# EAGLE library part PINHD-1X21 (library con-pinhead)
PIN HEADER
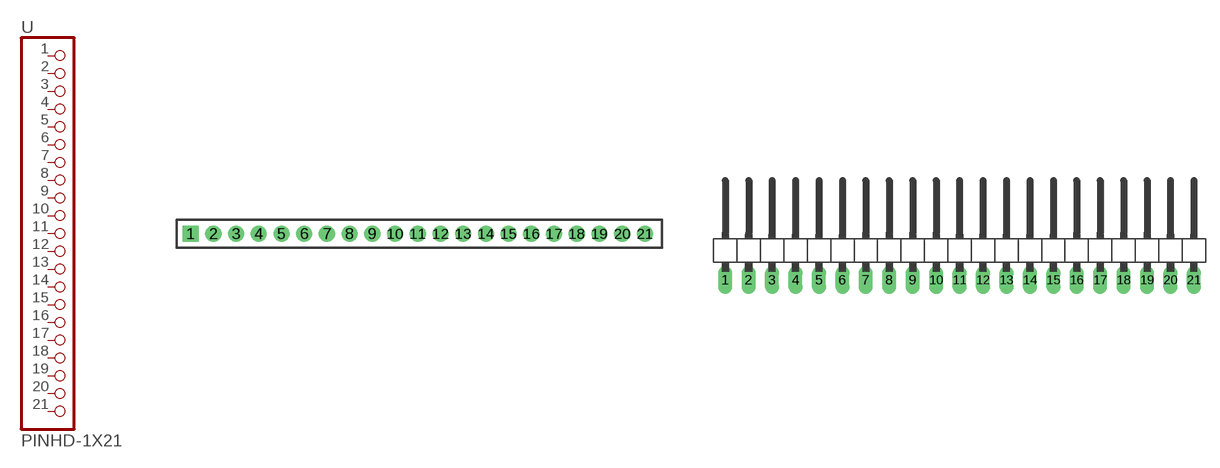
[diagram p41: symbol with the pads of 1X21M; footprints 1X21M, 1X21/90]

Designator prefix -

## PINHD-1X21_2.00  [1X21M]
1  1  pas
2  2  pas
3  3  pas
4  4  pas
5  5  pas
6  6  pas
7  7  pas
8  8  pas
9  9  pas
10  10  pas
11  11  pas
12  12  pas
13  13  pas
14  14  pas
15  15  pas
16  16  pas
17  17  pas
18  18  pas
19  19  pas
20  20  pas
21  21  pas

## PINHD-1X21_2.54-90°  [1X21/90]
Pads as for 1X21M

## PINHD-1X21_2.54  [1X21]
Pads as for 1X21M

## PINHD-1X21_2.54-SMD  [1X21SMD]
Pads as for 1X21M

## PINHD-1X21_2.54-SMD-90°  [1X21SMD/90]
Pads as for 1X21M

## Footprint 1X21M (pad centres in mm)
PIN HEADER - 2
drill 0.914 square: 1 -19,0
drill 0.914: 2 -17,0; 3 -15,0; 4 -13,0; 5 -11,0; 6 -9,0; 7 -7,0; 8 -5,0; 9 -3,0; 10 -1,0; 11 1,0; 12 3,0; 13 5,0; 14 7,0; 15 9,0; 16 11,0; 17 13,0; 18 15,0; 19 17,0; 20 19,0; 21 21,0

## Footprint 1X21/90 (pad centres in mm)
PIN HEADER - 2.54 90°
drill 1.016 long: 1 -24.13,-3.81; 2 -21.59,-3.81; 3 -19.05,-3.81; 4 -16.51,-3.81; 5 -13.97,-3.81; 6 -11.43,-3.81; 7 -8.89,-3.81; 8 -6.35,-3.81; 9 -3.81,-3.81; 10 -1.27,-3.81; 11 1.27,-3.81; 12 3.81,-3.81; 13 6.35,-3.81; 14 8.89,-3.81; 15 11.43,-3.81; 16 13.97,-3.81; 17 16.51,-3.81; 18 19.05,-3.81; 19 21.59,-3.81; 20 24.13,-3.81; 21 26.67,-3.81

## Footprint 1X21 (pad centres in mm)
PIN HEADER - 2.54
drill 1.016 long: 1 -24.13,0; 2 -21.59,0; 3 -19.05,0; 4 -16.51,0; 5 -13.97,0; 6 -11.43,0; 7 -8.89,0; 8 -6.35,0; 9 -3.81,0; 10 -1.27,0; 11 1.27,0; 12 3.81,0; 13 6.35,0; 14 8.89,0; 15 11.43,0; 16 13.97,0; 17 16.51,0; 18 19.05,0; 19 21.59,0; 20 24.13,0; 21 26.67,0

## Footprint 1X21SMD (pad centres in mm)
PIN HEADER - SMD
smd 1.016 x 3.302: 1 -1.27,1.27; 2 1.27,-1.27; 3 3.81,1.27; 4 6.35,-1.27; 5 8.89,1.27; 6 11.43,-1.27; 7 13.97,1.27; 8 16.51,-1.27; 9 19.05,1.27; 10 21.59,-1.27; 11 24.13,1.27; 12 26.67,-1.27; 13 29.21,1.27; 14 31.75,-1.27; 15 34.29,1.27; 16 36.83,-1.27; 17 39.37,1.27; 18 41.91,-1.27; 19 44.45,1.27; 20 46.99,-1.27; 21 49.53,1.27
